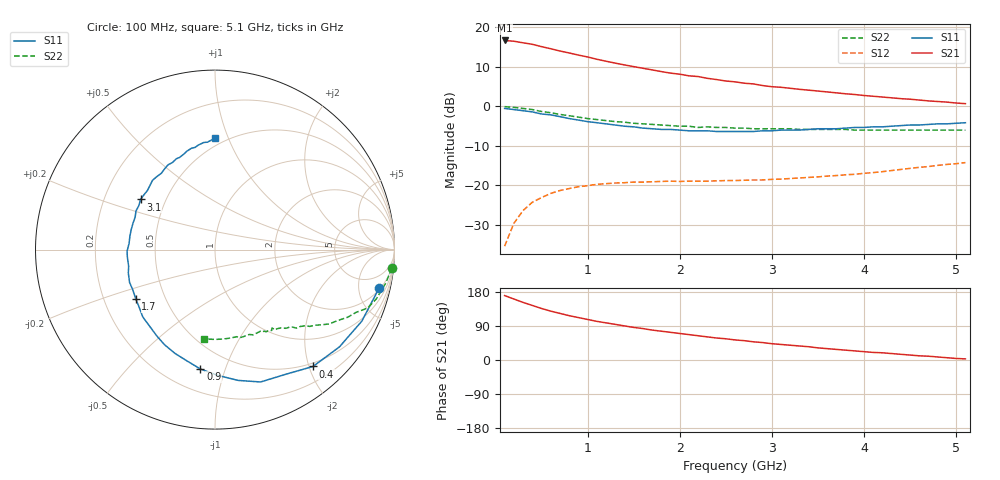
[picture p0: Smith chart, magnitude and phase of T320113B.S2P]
!AT-32011
!S and NOISE PARAMETERS at Vce=2.7 V  Ic=2mA.  LAST UPDATED 01-05-95
# ghz s ma r 50
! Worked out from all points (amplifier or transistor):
!   51 points, 100 MHz to 5.1 GHz, reference 50 ohm
!   highest |S21| = 16.7 dB at 100 MHz (marker M1)
!   |S21| within 3 dB of that: start of sweep to 766.8 MHz
!   unconditionally stable (mu >= 1): 2.388 GHz to 5.082 GHz
!   at 900 MHz: K = 0.39, MSG = 16.7 dB, |S12| = -20.4 dB
!   at 2.6 GHz: K = 1.07, MAG = 10.9 dB, |S12| = -18.8 dB
!   at 5.1 GHz: K = 1.00, MSG = 7.5 dB, |S12| = -14.2 dB
!   lowest NFmin = 0.57 dB at 500 MHz
!   S11 on the Smith chart (normalised r, x): 100 MHz: 2.25, -8.17; 400 MHz: 0.44, -2.07; 900 MHz: 0.34, -0.82; 1.7 GHz: 0.34, -0.26; 3.1 GHz: 0.36, +0.27; 5.1 GHz: 0.44, +0.90
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0.1  0.94 -13.0  6.81 170.0  0.017 82.0  0.99 -6.0
0.2  0.91 -26.0  6.66 161.0  0.033 75.0  0.97 -11.0
0.3  0.88 -38.0  6.36 152.0  0.048 68.0  0.94 -17.0
0.4  0.85 -50.0  6.09 144.0  0.061 62.0  0.91 -21.0
0.5  0.8 -60.0  5.69 136.0  0.07 57.0  0.86 -24.0
0.6  0.78 -71.0  5.35 129.0  0.079 52.0  0.83 -27.0
0.8  0.7 -89.0  4.73 117.0  0.091 44.0  0.76 -33.0
0.9  0.67 -97.0  4.45 112.0  0.096 41.0  0.73 -35.0
1  0.64 -104.0  4.21 107.0  0.099 39.0  0.7 -37.0
1.1  0.62 -111.0  3.94 102.0  0.103 37.0  0.68 -39.0
1.3  0.58 -124.0  3.52 94.0  0.107 33.0  0.64 -42.0
1.5  0.55 -137.0  3.18 86.0  0.11 30.0  0.61 -45.0
1.7  0.52 -148.0  2.89 79.0  0.111 28.0  0.59 -48.0
1.8  0.51 -154.0  2.75 76.0  0.112 28.0  0.58 -49.0
2.1  0.49 -169.0  2.43 67.0  0.113 27.0  0.56 -53.0
2.2  0.49 -175.0  2.38 64.0  0.113 27.0  0.54 -54.0
2.4  0.48 176.0  2.18 58.0  0.114 27.0  0.54 -57.0
2.6  0.48 167.0  2.04 53.0  0.115 28.0  0.53 -59.0
3.1  0.5 146.0  1.74 41.0  0.12 30.0  0.52 -65.0
3.5  0.52 132.0  1.56 32.0  0.128 33.0  0.51 -70.0
4.3  0.56 108.0  1.28 17.0  0.154 38.0  0.5 -82.0
5.1  0.62 90.0  1.08 3.0  0.194 37.0  0.5 -97.0
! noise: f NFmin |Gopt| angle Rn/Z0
0.5  0.57  0.69  22  0.3
0.9  0.78  0.6  51  0.25
1.8  1.25  0.42  117  0.14
2.4  1.57  0.44  159  0.08
